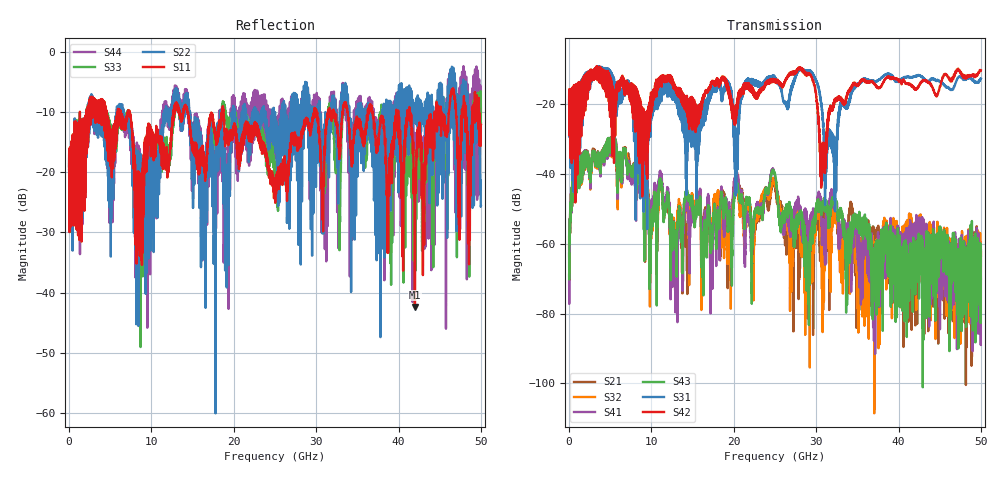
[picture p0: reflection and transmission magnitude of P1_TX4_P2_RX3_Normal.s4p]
!Keysight Technologies,N5225B,MY57041031,A.13.20.10
!Date: Friday, May 31, 2019 11:31:48
!Correction: S11(Full 4 Port(1,2,3,4))
!S12(Full 4 Port(1,2,3,4))
!S13(Full 4 Port(1,2,3,4))
!S14(Full 4 Port(1,2,3,4))
!S21(Full 4 Port(1,2,3,4))
!S22(Full 4 Port(1,2,3,4))
!S23(Full 4 Port(1,2,3,4))
!S24(Full 4 Port(1,2,3,4))
!S31(Full 4 Port(1,2,3,4))
!S32(Full 4 Port(1,2,3,4))
!S33(Full 4 Port(1,2,3,4))
!S34(Full 4 Port(1,2,3,4))
!S41(Full 4 Port(1,2,3,4))
!S42(Full 4 Port(1,2,3,4))
!S43(Full 4 Port(1,2,3,4))
!S44(Full 4 Port(1,2,3,4))
!S4P File: Measurements: <S11,S12,S13,S14>,
!<S21,S22,S23,S24>,
!<S31,S32,S33,S34>,
!<S41,S42,S43,S44>:
# Hz S  dB  R 50.0
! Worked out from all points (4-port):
!   5000 points, 10 MHz to 50 GHz, reference 50 ohm
!   strongest paths, dB at 10 MHz, 12.51 GHz, 25.01 GHz, 37.51 GHz, 50 GHz:
!     S42: -19.4, -14.2, -13.2, -15.2, -10.2
!     S31: -19.5, -17.9, -13.0, -13.1, -12.6
!     S43: -62.8, -59.9, -39.9, -66.3, -69.9
!     S41: -68.8, -58.6, -40.5, -58.1, -63.1
!     S32: -58.0, -57.9, -42.5, -64.8, -62.4
!     S21: -60.3, -68.1, -43.3, -56.7, -61.8
!   lowest |S11| = -42.4 dB at 41.99 GHz (marker M1), VSWR 1.02, Z = 50.6 - j0.43 ohm
!   |S11| at or under -10 dB: 7.334 GHz to 12.7 GHz (5.364 GHz wide, 53.6 % of centre); 14.41 GHz to 18.57 GHz (4.157 GHz wide, 25.2 % of centre); 18.74 GHz to 29.76 GHz (11.02 GHz wide, 45.4 % of centre)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
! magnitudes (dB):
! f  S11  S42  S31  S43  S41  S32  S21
! 10 MHz  -19.5  -19.4  -19.5  -62.8  -68.8  -58.0  -60.3
! 820 MHz  -17.8  -17.2  -18.5  -37.6  -37.4  -37.8  -37.5
! 4.97 GHz  -13.0  -15.5  -10.3  -30.3  -30.6  -30.7  -30.6
! 12.95 GHz  -8.6  -15.7  -19.3  -59.5  -66.7  -56.3  -63.6
! 20.3 GHz  -14.0  -20.6  -34.2  -43.2  -40.1  -43.3  -40.6
! 41.99 GHz  -42.4  -15.5  -12.0  -71.2  -56.8  -57.7  -58.7
! 50 GHz  -12.1  -10.2  -12.6  -69.9  -63.1  -62.4  -61.8
